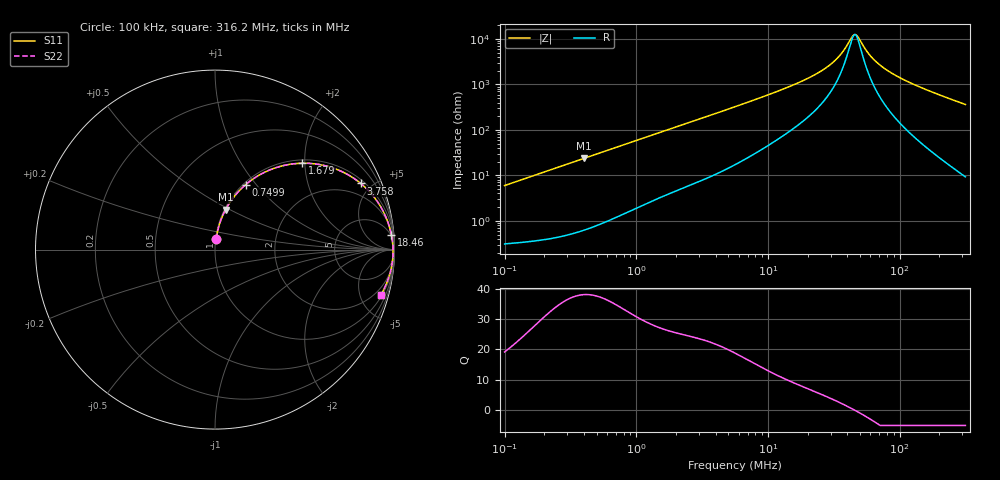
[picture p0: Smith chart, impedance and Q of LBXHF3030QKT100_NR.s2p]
! LBXHF3030QKT100_NR  S-PARAMETER MODEL  ( General Type )
! Model Generated by TAIYO YUDEN Corporation (http://www.ty-top.com)
! Version 1.0
! TAIYO YUDEN Control No. 210113NI43SB-FBB
! Copyright(c) 2021 TAIYO YUDEN CO.,LTD. All Rights Reserved.
! Product Description (link to TY-COMPAS)
! https://ds.yuden.co.jp/TYCOMPAS/or/detail?pn=LBXHF3030QKT100MNR&u=M
! Products Name : Inductors
! Characteristics :
!  Inductance : 10 uH , SRF(min) : 20 MHz , DC Resistance(max) : 0.228 Ohm
!  Rated Current : Saturation :760 mA , Temp Rise : 750 mA
!  Case Size : 3.0 x 3.0 / 0.118 x 0.118 [mm/inch] , Thickness : 1.5 / 0.059 [mm/inch]
!  (Conditions: Temperature = 25 degC , DC Bias Current/Voltage = 0A / 0V)
! External Node Assignments :
!  1  o---GGG---o  2
! GND o---------o GND
! Frequency Range : 0.1MHz  -  316.199832MHz  [ 402 STEP ]
# MHz S RI R 50
! Freq[MHz].  S11 Real  S11 Imag  S21 Real  S21 Imag  S12 Real  S12 Imag  S22 Real  S22 Imag
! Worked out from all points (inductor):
!   401 points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, 100 kHz to 316.2 MHz, reference 50 ohm
!   read as one part in series: L = 9.48 uH near 104.1 kHz
!   highest Q = 38 at 401.6 kHz (marker M1), where L = 9.41 uH
!   self-resonance near 45.71 MHz
!   S11 on the Smith chart (normalised r, x): 100 kHz: 1.01, +0.12; 749.9 kHz: 1.03, +0.88; 1.679 MHz: 1.07, +1.95; 3.758 MHz: 1.19, +4.31; 18.46 MHz: 4, +24; 316.2 MHz: 1.19, -7.25
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0.1  0.00662 0.0591  0.9934 -0.0591  0.9934 -0.0591  0.00662 0.0591
0.385695  0.0546 0.2144  0.9454 -0.2144  0.9454 -0.2144  0.0546 0.2144
0.401553  0.0587 0.2222  0.9413 -0.2222  0.9413 -0.2222  0.0587 0.2222
0.749878  0.1701 0.3613  0.8299 -0.3613  0.8299 -0.3613  0.1701 0.3613
1.487603  0.4304 0.4771  0.5696 -0.4771  0.5696 -0.4771  0.4304 0.4771
1.678752  0.4871 0.4813  0.5129 -0.4813  0.5129 -0.4813  0.4871 0.4813
2.412597  0.6529 0.4561  0.3471 -0.4561  0.3471 -0.4561  0.6529 0.4561
3.758225  0.8121 0.3687  0.1879 -0.3687  0.1879 -0.3687  0.8121 0.3687
5.623165  0.9006 0.2738  0.0994 -0.2738  0.0994 -0.2738  0.9006 0.2738
18.45972  0.983 0.0798  0.017 -0.0798  0.017 -0.0798  0.983 0.0798
21.68824  0.986 0.0634  0.014 -0.0634  0.014 -0.0634  0.986 0.0634
27.06907  0.9889 0.043  0.0111 -0.043  0.0111 -0.043  0.9889 0.043
32.45058  0.9906 0.0276  0.00943 -0.0276  0.00943 -0.0276  0.9906 0.0276
37.36559  0.9914 0.0162  0.00858 -0.0162  0.00858 -0.0162  0.9914 0.0162
43.90066  0.992 0.00331  0.00799 -0.00331  0.00799 -0.00331  0.992 0.00331
45.70575  0.9921 0.000109  0.0079 -0.000109  0.0079 -0.000109  0.9921 0.000109
48.5535  0.9922 -0.0047  0.00782 0.0047  0.00782 0.0047  0.9922 -0.0047
55.90748  0.9921 -0.0161  0.00785 0.0161  0.00785 0.0161  0.9921 -0.0161
63.09128  0.9919 -0.0261  0.00813 0.0261  0.00813 0.0261  0.9919 -0.0261
83.65039  0.9902 -0.0511  0.00984 0.0511  0.00984 0.0511  0.9902 -0.0511
141.2425  0.9808 -0.1095  0.0192 0.1095  0.0192 0.1095  0.9808 -0.1095
316.1998  0.9238 -0.2529  0.0762 0.2529  0.0762 0.2529  0.9238 -0.2529
